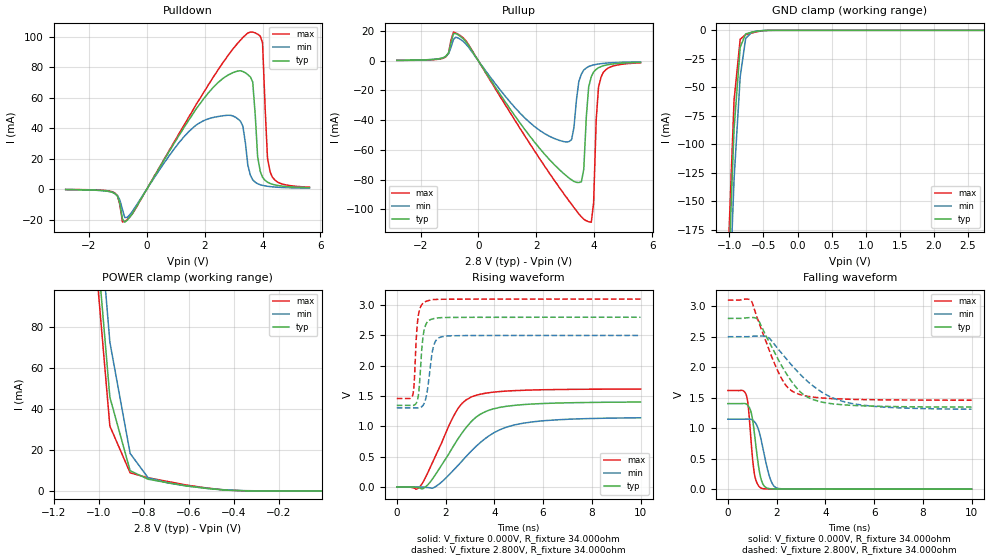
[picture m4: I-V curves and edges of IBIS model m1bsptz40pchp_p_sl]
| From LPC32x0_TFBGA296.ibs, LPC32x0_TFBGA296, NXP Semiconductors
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| |   Rev 0.20 IBIS Model Design Automation Generation   |
| |   N O N - S I L I C O N   C O R R E L A T E D   |
| |   This IBIS [Model] is pre-Beta tactical support   |
| |  Note: this IBIS [Model] contains clamp curves generated   |
| |   through simulation which should not be relied upon   |
| mem1bsptz40pchp
|   Bidirectional Pad 2.8
|   3state Output
|   Plain Input
|   1ns Slew Rate control
|   CMOS
| Plain input Mode (p1=0, p2=1)
[Model]   m1bsptz40pchp_p_sl | of mem1bsptz40pchp
Model_type   I/O
Polarity   Non-Inverting
Enable   Active-Low
|  Reciever Thresholds
Vinl   = 0.36V
Vinh   = 0.84V
| AC Test Load Conditions
Vref   = 0
Cref   = 1.2e-11
Rref   = 1000000000
Vmeas   = 0.6
| [Process Range]   typical   min   max
| C_comp edge width   400.000ps   400.000ps   400.000ps
| C_comp Tstrobe   40.000fs   40.000fs   40.000fs
C_comp   2.023pF   1.952pF   2.110pF
[Temperature Range]   25   125   -40
[Voltage Range]   2.80V   2.50V   3.10V
[GND Clamp Reference]   0.00V   0.00V   0.00V
[Pulldown Reference]   0.00V   0.00V   0.00V
[POWER Clamp Reference]   2.80V   2.50V   3.10V
[Pullup Reference]   2.80V   2.50V   3.10V
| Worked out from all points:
|   slope of the pulldown table from 0 to 0.42 V, typ, clamps not added: 30.8 ohm
|   slope of the pullup table from 0 to 0.42 V, typ, clamps not added: 32.8 ohm
|   GND clamp passes 1 mA (typ) near -0.62 V on its own axis
|   POWER clamp passes 1 mA (typ) near -0.50 V on its own axis
|   rising waveform, V_fixture 0.000V, R_fixture 34.000ohm: 20-80 % time 1.45ns typ, 1.87ns min, 1.14ns max; typ from 0 V to 1.4 V
|   falling waveform, V_fixture 0.000V, R_fixture 34.000ohm: 20-80 % time 278ps typ, 392ps min, 211ps max; typ from 1.4 V to 0 V
|   rising waveform, V_fixture 2.800V, R_fixture 34.000ohm: 20-80 % time 169ps typ, 240ps min, 142ps max; typ from 1.34 V to 2.8 V
|   falling waveform, V_fixture 2.800V, R_fixture 34.000ohm: 20-80 % time 1.3ns typ, 1.9ns min, 1.01ns max; typ from 2.8 V to 1.35 V
[GND Clamp]
| ref voltage   0.00V   0.00V   0.00V
|   Voltage   I(typ)   I(min)   I(max)
-2.8V     -3.643A    -3.653A    -3.644A
-1.01V    -211.8mA   -255.9mA   -186.6mA
-930mV    -86.59mA   -130.6mA   -61.22mA
-840mV    -14.8mA    -40.63mA   -7.788mA
-760mV    -3.159mA   -7.066mA   -3.782mA
-670mV    -1.57mA    -1.656mA   -2.327mA
-500mV    -164.9uA   -160.9uA   -333.4uA
2.73V     191.3pA    5.77uA     169pA
[Power Clamp]   | Vtable = Vcc - Vpad
| ref voltage   2.80V   2.50V   3.10V
|   Voltage   I(typ)   I(min)   I(max)
-2.82V    3.531A     3.518A     3.546A
-1.03V    149.7mA    178.4mA    134.4mA
-950mV    45.7mA     72.61mA    31.64mA
-860mV    9.848mA    18.29mA    8.836mA
-780mV    5.694mA    6.392mA    6.4mA
-690mV    3.927mA    3.849mA    4.543mA
-610mV    2.433mA    2.409mA    2.865mA
-440mV    389uA      533.2uA    433.4uA
-350mV    49.46uA    132.2uA    33.93uA
-10mV     426.3pA    7.713nA    250.7pA
[Pulldown]
| ref voltage   0.00V   0.00V   0.00V
|   Voltage   I(typ)   I(min)   I(max)
-2.8V     -319.4uA   -345.4uA   -253.4uA
-1.18V    -2.16mA    -2.186mA   -1.788mA
-670mV    -20.32mA   -18.55mA   -19.96mA
2.13V     63.18mA    46.12mA    68.49mA
3.24V     77.6mA     44.48mA    97.75mA
3.58V     73.59mA    9.104mA    103mA
3.66V     70.25mA    6.083mA    103mA
3.83V     21.2mA     3.504mA    101.6mA
4V        7.749mA    2.422mA    96.02mA
4.17V     4.517mA    1.836mA    20.5mA
4.26V     3.724mA    1.635mA    11.42mA
5.62V     951.1uA    582.3uA    1.268mA
[Pullup]   | Vtable = Vcc - Vpad
| ref voltage   2.80V   2.50V   3.10V
|   Voltage   I(typ)   I(min)   I(max)
-2.82V    285.5uA    305.8uA    228.3uA
-520mV    14.78mA    13mA       15.38mA
2.79V     -73.2mA    -53.56mA   -85.24mA
3.22V     -80.21mA   -53.04mA   -96.65mA
3.47V     -82mA      -13.93mA   -103.2mA
3.64V     -72.97mA   -6.254mA   -106.7mA
3.81V     -17.59mA   -3.875mA   -108.5mA
3.9V      -10.76mA   -3.236mA   -108.7mA
3.98V     -7.521mA   -2.772mA   -95.82mA
4.07V     -5.763mA   -2.42mA    -39.47mA
4.24V     -3.891mA   -1.925mA   -10.83mA
5.6V      -1.047mA   -713.1uA   -1.374mA
[Ramp]
R_load   = 34.000ohm
|   dV/dt(typ)   dV/dt(min)   dV/dt(max)
dV/dt_r   970.587mV/1.300ns   805.818mV/1.660ns   1.110V/1.030ns
dV/dt_f   1.001V/1.125ns   838.617mV/1.635ns   1.124V/885.000ps
[Rising Waveform]  | cubic spline decimation from 2001 points
V_fixture   = 0.000V
R_fixture   = 34.000ohm
|   Time   V(typ)   V(min)   V(max)
0s        4.315nV    140.2nV    2.475nV
810ps     -7.213mV   186uV      -37.67mV
975ps     -22.57mV   -1.932mV   16.38mV
1.2ns     7.442mV    -7.991mV   172.6mV
1.54ns    174.7mV    -7.819mV   467.7mV
2.43ns    741.2mV    319.4mV    1.24V
3.095ns   1.093V     606.7mV    1.49V
4ns       1.291V     896.3mV    1.565V
5.185ns   1.358V     1.051V     1.594V
10ns      1.4V       1.141V     1.615V
[Falling Waveform]  | cubic spline decimation from 2001 points
V_fixture   = 0.000V
R_fixture   = 34.000ohm
|   Time   V(typ)   V(min)   V(max)
0s        1.403V     1.147V     1.617V
750ps     1.398V     1.148V     1.55V
835ps     1.369V     1.149V     1.369V
955ps     1.259V     1.143V     785mV
1.09ns    918.2mV    1.107V     253.4mV
1.26ns    377.7mV    973mV      55.2mV
1.375ns   150.1mV    793.8mV    16.17mV
1.74ns    6.839mV    170.1mV    1.944mV
2.055ns   1.816mV    13.85mV    1.102mV
10ns      7.546uV    12.11uV    6.875uV
[Rising Waveform]  | cubic spline decimation from 2001 points
V_fixture   = 2.800V
V_fixture_min = 2.500V
V_fixture_max = 3.100V
R_fixture   = 34.000ohm
|   Time   V(typ)   V(min)   V(max)
0s        1.345V     1.305V     1.458V
660ps     1.345V     1.305V     1.523V
720ps     1.351V     1.305V     1.754V
825ps     1.403V     1.303V     2.602V
910ps     1.595V     1.304V     2.881V
1.07ns    2.456V     1.342V     3.029V
1.19ns    2.676V     1.458V     3.06V
1.51ns    2.777V     2.324V     3.092V
1.825ns   2.793V     2.475V     3.096V
10ns      2.8V       2.5V       3.1V
[Falling Waveform]  | cubic spline decimation from 2001 points
V_fixture   = 2.800V
V_fixture_min = 2.500V
V_fixture_max = 3.100V
R_fixture   = 34.000ohm
|   Time   V(typ)   V(min)   V(max)
0s        2.8V       2.5V       3.1V
965ps     2.814V     2.505V     3.084V
1.27ns    2.76V      2.512V     2.737V
1.67ns    2.434V     2.484V     2.309V
2.13ns    2.08V      2.266V     1.872V
2.46ns    1.857V     2.109V     1.666V
2.865ns   1.64V      1.926V     1.564V
3.98ns    1.418V     1.561V     1.492V
5.045ns   1.375V     1.408V     1.473V
10ns      1.346V     1.311V     1.459V
